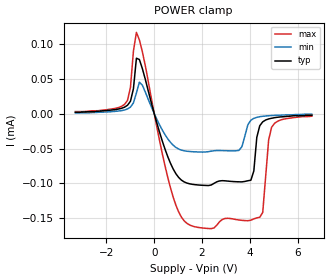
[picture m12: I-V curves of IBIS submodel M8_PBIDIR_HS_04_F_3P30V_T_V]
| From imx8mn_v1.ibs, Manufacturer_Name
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| Submodel
[Submodel]  M8_PBIDIR_HS_04_F_3P30V_T_V
Submodel_type Dynamic_clamp
[POWER Clamp]
| Voltage   I(typ)   I(min)   I(max)
-3.3V     1.907uA    953.7nA    2.861uA
-1.241V   9.179uA    5.181uA    13.15uA
-993.1mV  17.73uA    9.307uA    37.7uA
-744.8mV  79.21uA    29.51uA    116.2uA
910.3mV   -86.2uA    -48.48uA   -131.3uA
2.39V     -102.1uA   -53.72uA   -164.7uA
3.548V    -97.65uA   -52.63uA   -152.3uA
4.045V    -95.34uA   -9.513uA   -152.5uA
4.417V    -17.34uA   -4.47uA    -148.4uA
4.541V    -11.8uA    -3.854uA   -141.4uA
4.914V    -6.676uA   -2.762uA   -19.5uA
6.6V      -2.384uA   -953.7nA   -3.735uA
